FUNCTION F_ConvByteArrToBitArr : BOOL
VAR_INPUT
END_VAR
VAR_IN_OUT
	nSrcBytes			: ARRAY[*] OF BYTE;		// Source Array of Byte
	nDestBits			: ARRAY[*] OF BOOL;		// Destination Array of BOOL
END_VAR
VAR
	nLowerBoundSrc		: DINT;					// lowest index of source-array
	nUpperBoundSrc		: DINT;					// highest index of source-array
	nCntSrc				: DINT;					// number of elements in source-array
	
	nLowerBoundDest		: DINT;					// lowest index of destination-array
	nUpperBoundDest		: DINT;					// highest index of destination-array
	nCntDest			: DINT;					// number of elements in destination-array
	
	nIdx				: DINT;					// loop-index
END_VAR

IF nSrcBytes <> 0 AND nDestBits <> 0 THEN
	
	// get array dimensions
	nLowerBoundSrc := LOWER_BOUND(nSrcBytes, 1);
	nUpperBoundSrc := UPPER_BOUND(nSrcBytes, 1);
	nCntSrc := nUpperBoundSrc - nLowerBoundSrc + 1;
	
	nLowerBoundDest := LOWER_BOUND(nDestBits, 1);
	nUpperBoundDest := UPPER_BOUND(nDestBits, 1);
	nCntDest := nUpperBoundDest - nLowerBoundDest + 1;
	
	// check if destination is big enough
	IF nCntDest >= 8 * nCntSrc THEN
		FOR nIdx := 0 TO nCntSrc - 1 DO
			//nDestBits[(i-1)*8+1]
			nDestBits[nLowerBoundDest + nidx * 8] := nSrcBytes[nLowerBoundSrc + nIdx].0;
			nDestBits[nLowerBoundDest + nidx * 8 + 1] := nSrcBytes[nLowerBoundSrc + nIdx].1;
			nDestBits[nLowerBoundDest + nidx * 8 + 2] := nSrcBytes[nLowerBoundSrc + nIdx].2;
			nDestBits[nLowerBoundDest + nidx * 8 + 3] := nSrcBytes[nLowerBoundSrc + nIdx].3;
			nDestBits[nLowerBoundDest + nidx * 8 + 4] := nSrcBytes[nLowerBoundSrc + nIdx].4;
			nDestBits[nLowerBoundDest + nidx * 8 + 5] := nSrcBytes[nLowerBoundSrc + nIdx].5;
			nDestBits[nLowerBoundDest + nidx * 8 + 6] := nSrcBytes[nLowerBoundSrc + nIdx].6;
			nDestBits[nLowerBoundDest + nidx * 8 + 7] := nSrcBytes[nLowerBoundSrc + nIdx].7;
		END_FOR
		
		F_ConvByteArrToBitArr := TRUE;
	ELSE
		F_ConvByteArrToBitArr := FALSE;
	END_IF

ELSE
	F_ConvByteArrToBitArr := FALSE;
END_IF

END_FUNCTION
